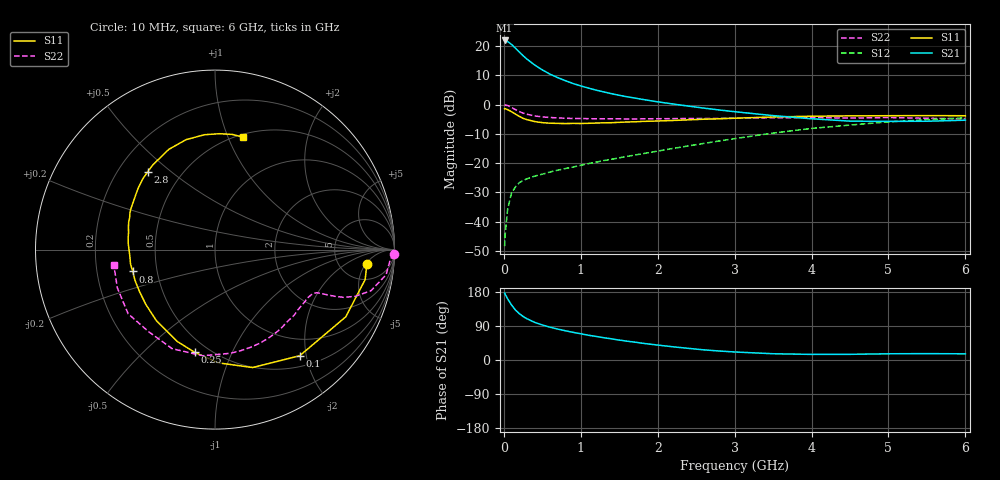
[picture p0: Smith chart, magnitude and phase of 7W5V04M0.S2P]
! Infineon Technologies  Discrete & RF Semiconductors
! BFS17W
! Si NPN RF Bipolar Junction Transistor in SOT323
! VCE = 5 V  IC = 4 mA
! Common Emitter S-Parameters:  August  1999
# GHz  S  MA  R  50
!  f  S11  S21  S12  S22
! GHz  MAG  ANG  MAG  ANG  MAG  ANG  MAG  ANG
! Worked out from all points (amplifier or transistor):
!   36 points, 10 MHz to 6 GHz, reference 50 ohm
!   highest |S21| = 21.9 dB at 10 MHz (marker M1)
!   |S21| within 3 dB of that: start of sweep to 164.8 MHz
!   unconditionally stable (mu >= 1): 639.2 MHz to 2.647 GHz; 4.444 GHz to end of sweep
!   at 250 MHz: K = 0.52, MSG = 21.4 dB, |S12| = -26.0 dB
!   at 1.4 GHz: K = 1.24, MAG = 8.3 dB, |S12| = -18.7 dB
!   at 6 GHz: K = 1.07, MAG = -2.0 dB, |S12| = -4.5 dB
!   S11 on the Smith chart (normalised r, x): 10 MHz: 9, -5; 100 MHz: 0.68, -1.88; 250 MHz: 0.42, -0.73; 800 MHz: 0.36, -0.11; 2.8 GHz: 0.32, +0.42; 6 GHz: 0.53, +1.14
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0.01  0.8503 -5.4  12.51 176.6  0.0038 86.6  0.9969 -1.3
0.02  0.8531 -11.3  12.4 172.3  0.0067 83.8  0.9776 -3.4
0.05  0.8192 -27.2  11.99 161.1  0.0165 76.3  0.9633 -8.4
0.1  0.7566 -51.4  10.69 145.2  0.0308 65.2  0.8982 -14.8
0.15  0.6898 -72.3  9.26 132.1  0.0391 57.2  0.8218 -18.5
0.2  0.6315 -88.2  7.962 122.5  0.0462 53.2  0.7628 -20.4
0.25  0.5834 -101.2  6.871 114.9  0.0503 49.3  0.7164 -21.3
0.3  0.5533 -112.3  6.011 108.9  0.0539 48.8  0.6844 -21.8
0.4  0.5138 -129.3  4.765 99.4  0.0599 47.7  0.6412 -22.4
0.5  0.4918 -141.6  3.925 92.4  0.0646 48.2  0.6174 -22.9
0.6  0.4815 -150.8  3.32 86.6  0.0704 49.8  0.6027 -23.8
0.8  0.4743 -165.1  2.564 77.1  0.0808 53.3  0.585 -26.7
0.9  0.4775 -170.3  2.297 73.0  0.0857 54.9  0.5801 -28.2
1.1  0.4791 179.9  1.918 65.3  0.0981 57.5  0.5749 -32.1
1.3  0.4884 172.0  1.648 58.8  0.1106 60.2  0.5709 -36.5
1.6  0.505 162.2  1.363 49.7  0.1302 63.1  0.5691 -43.4
2.2  0.5356 145.9  1.025 34.8  0.1783 66.9  0.5763 -59.0
2.8  0.5734 130.9  0.81 23.7  0.2389 67.4  0.5812 -76.0
3.5  0.6151 114.7  0.649 16.5  0.3264 63.7  0.5956 -96.6
4.5  0.6427 95.2  0.522 15.0  0.4474 51.9  0.5882 -129.1
5.5  0.6489 81.3  0.52 16.8  0.5528 38.9  0.5844 -158.5
6  0.6454 75.9  0.542 16.3  0.5938 32.6  0.5704 -171.5
